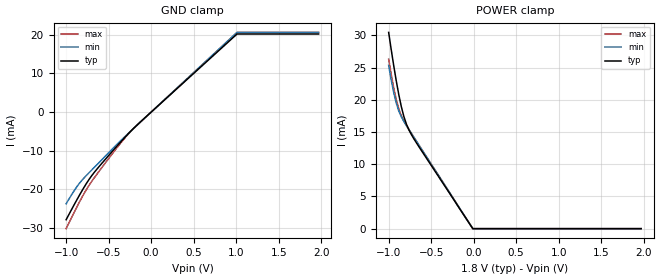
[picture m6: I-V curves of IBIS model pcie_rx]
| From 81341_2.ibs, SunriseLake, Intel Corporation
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[Model]   pcie_rx
Model_type   Input
Polarity   Non-Inverting
Vinl = -0.11
Vinh = 0.11
|   typ   min   max
C_comp   1.0308pF   1.019pF   1.0309pF
[Voltage Range]   1.800V   1.710V   1.890V
[Temperature Range]   60.0   105.0   0.0
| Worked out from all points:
|   GND clamp passes 1 mA (typ) near -0.05 V on its own axis
|   POWER clamp passes 1 mA (typ) near -0.06 V on its own axis
[GND Clamp]
|   Voltage   I(typ)   I(min)   I(max)
-1V       -27.81mA   -23.69mA   -30.12mA
-910mV    -24.11mA   -20.45mA   -26.09mA
-850mV    -21.72mA   -18.56mA   -23.5mA
-760mV    -18.38mA   -16.33mA   -19.95mA
-700mV    -16.45mA   -14.98mA   -17.93mA
-460mV    -10.22mA   -9.629mA   -10.85mA
-280mV    -5.836mA   -5.728mA   -5.939mA
-130mV    -2.607mA   -2.651mA   -2.652mA
1.01V     20.18mA    20.6mA     20.58mA
1.97V     20.18mA    20.6mA     20.58mA
[POWER Clamp]
|   Voltage   I(typ)   I(min)   I(max)
-1V       30.46mA    25.35mA    26.31mA
-970mV    27.81mA    23.09mA    23.96mA
-940mV    25.27mA    21.09mA    21.83mA
-910mV    22.9mA     19.45mA    20.01mA
-880mV    20.75mA    18.23mA    18.57mA
-850mV    18.89mA    17.34mA    17.5mA
-820mV    17.37mA    16.62mA    16.69mA
-790mV    16.19mA    15.97mA    16mA
-730mV    14.54mA    14.73mA    14.74mA
-670mV    13.25mA    13.5mA     13.51mA
-10mV     0A         0A         0A
1.97V     0A         0A         0A
